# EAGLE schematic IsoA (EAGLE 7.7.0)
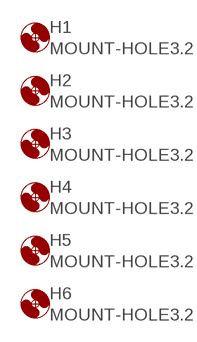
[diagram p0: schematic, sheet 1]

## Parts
H1  MOUNT-HOLE3.2  [3,2]
H2  MOUNT-HOLE3.2  [3,2]
H3  MOUNT-HOLE3.2  [3,2]
H4  MOUNT-HOLE3.2  [3,2]
H5  MOUNT-HOLE3.2  [3,2]
H6  MOUNT-HOLE3.2  [3,2]

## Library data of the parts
H1-H6 = holes:MOUNT-HOLE: MOUNTING HOLE with drill center marker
